FUNCTION "FC_GRP_51" : VOID
TITLE =GROUP =51
{ S7_language := '9(1) Angielski (Stany Zjednoczone)  11.01.2022  09:45:15' }
VERSION : 0.1


VAR_TEMP
  CL : "UDT_CABINET";	//CABINET LOCAL
  CR : "UDT_CABINET";	//CABINET REMOTE
  RelError : BOOL ;	//ERROR RELEASE
  RelErrorCL : BOOL ;	//ERROR RELEASE FROM CABINET LOCAL
  RelErrorCR : BOOL ;	//ERROR RELEASE FROM CABINET REMOTE
  RelControl : BOOL ;	//CONTROL RELEASE
  RelControlCL : BOOL ;	//CONTROL RELEASE FROM CABINET LOCAL
  RelControlCR : BOOL ;	//CONTROL RELEASE FROM CABINET REMOTE
  ErrorConfirm : BOOL ;	//ERROR CONFIRM
  AutoOn : BOOL ;	//AUTOMATIC ON
  AutoOff : BOOL ;	//AUTOMATIC OFF
  RelAuto : BOOL ;	//AUTOMATIC RELEASE
  LAMP_ON : BOOL ;
  TempSetpoint : REAL ;
END_VAR
BEGIN
NETWORK
TITLE =GLOBAL SIGNALS
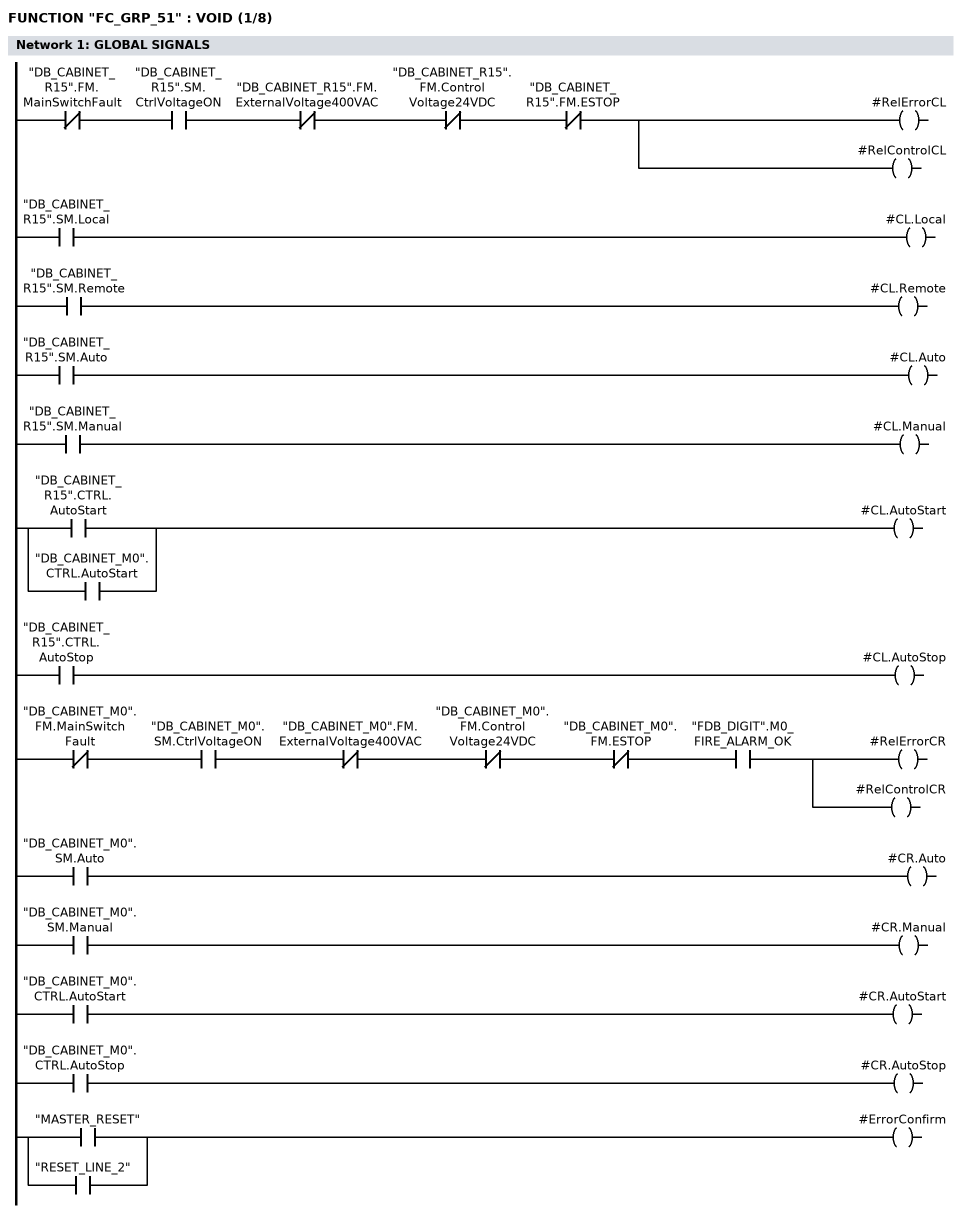
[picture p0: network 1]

//LOCAL
      UN    "DB_CABINET_R15".FM.MainSwitchFault;
      U     "DB_CABINET_R15".SM.CtrlVoltageON;
      UN    "DB_CABINET_R15".FM.ExternalVoltage400VAC;
      UN    "DB_CABINET_R15".FM.ControlVoltage24VDC;
      UN    "DB_CABINET_R15".FM.ESTOP;
      =     #RelErrorCL;
      =     #RelControlCL;

      U     "DB_CABINET_R15".SM.Local;
      =     #CL.Local;
      U     "DB_CABINET_R15".SM.Remote;
      =     #CL.Remote;
      U     "DB_CABINET_R15".SM.Auto;
      =     #CL.Auto;
      U     "DB_CABINET_R15".SM.Manual;
      =     #CL.Manual;
      U     "DB_CABINET_R15".CTRL.AutoStart;
      O     "DB_CABINET_M0".CTRL.AutoStart;
      =     #CL.AutoStart;
      U     "DB_CABINET_R15".CTRL.AutoStop;
      =     #CL.AutoStop;


//REMOTE

      UN    "DB_CABINET_M0".FM.MainSwitchFault;
      U     "DB_CABINET_M0".SM.CtrlVoltageON;
      UN    "DB_CABINET_M0".FM.ExternalVoltage400VAC;
      UN    "DB_CABINET_M0".FM.ControlVoltage24VDC;
//      UN    "DB_CABINET_M0".FM.ControlVoltage230VAC_MS
      UN    "DB_CABINET_M0".FM.ESTOP;
      U     "FDB_DIGIT".M0_FIRE_ALARM_OK;
      =     #RelErrorCR;
      =     #RelControlCR;

      U     "DB_CABINET_M0".SM.Auto;
      =     #CR.Auto;
      U     "DB_CABINET_M0".SM.Manual;
      =     #CR.Manual;
      U     "DB_CABINET_M0".CTRL.AutoStart;
      =     #CR.AutoStart;
      U     "DB_CABINET_M0".CTRL.AutoStop;
      =     #CR.AutoStop;


      U     "MASTER_RESET";
      O     "RESET_LINE_2";
      =     #ErrorConfirm;

NETWORK
TITLE =GLOBAL SIGNALS - GROUP GENERAL ERROR AND WARNING
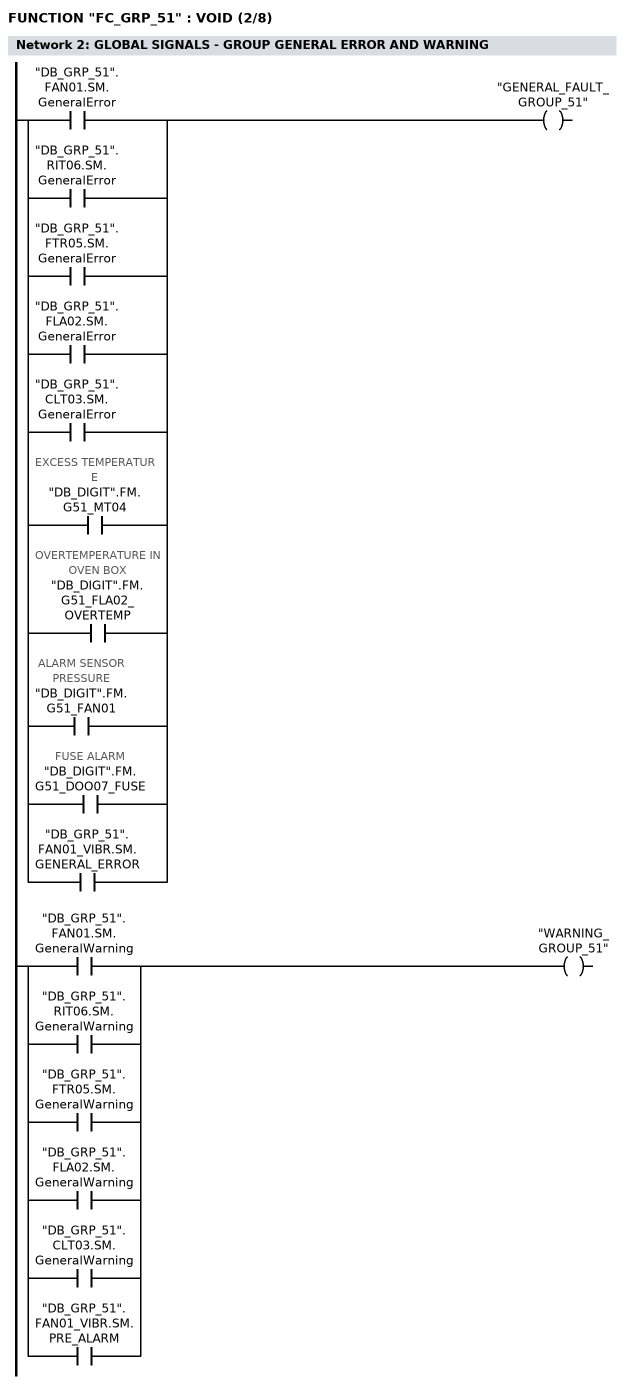
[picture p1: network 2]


      U     "DB_GRP_51".FAN01.SM.GeneralError;
      O     "DB_GRP_51".RIT06.SM.GeneralError;
      O     "DB_GRP_51".FTR05.SM.GeneralError;
      O     "DB_GRP_51".FLA02.SM.GeneralError;
      O     "DB_GRP_51".CLT03.SM.GeneralError;
      O     "DB_DIGIT".FM.G51_MT04; //EXCESS TEMPERATURE
      O     "DB_DIGIT".FM.G51_FLA02_OVERTEMP; //OVERTEMPERATURE IN OVEN BOX
      O     "DB_DIGIT".FM.G51_FAN01; //ALARM SENSOR PRESSURE
      O     "DB_DIGIT".FM.G51_DOO07_FUSE; //FUSE ALARM
      O     "DB_GRP_51".FAN01_VIBR.SM.GENERAL_ERROR;
      =     "GENERAL_FAULT_GROUP_51";

      U     "DB_GRP_51".FAN01.SM.GeneralWarning;
      O     "DB_GRP_51".RIT06.SM.GeneralWarning;
      O     "DB_GRP_51".FTR05.SM.GeneralWarning;
      O     "DB_GRP_51".FLA02.SM.GeneralWarning;
      O     "DB_GRP_51".CLT03.SM.GeneralWarning;
      O     "DB_GRP_51".FAN01_VIBR.SM.PRE_ALARM;
      =     "WARNING_GROUP_51";


NETWORK
TITLE =RELEASE CONTROL
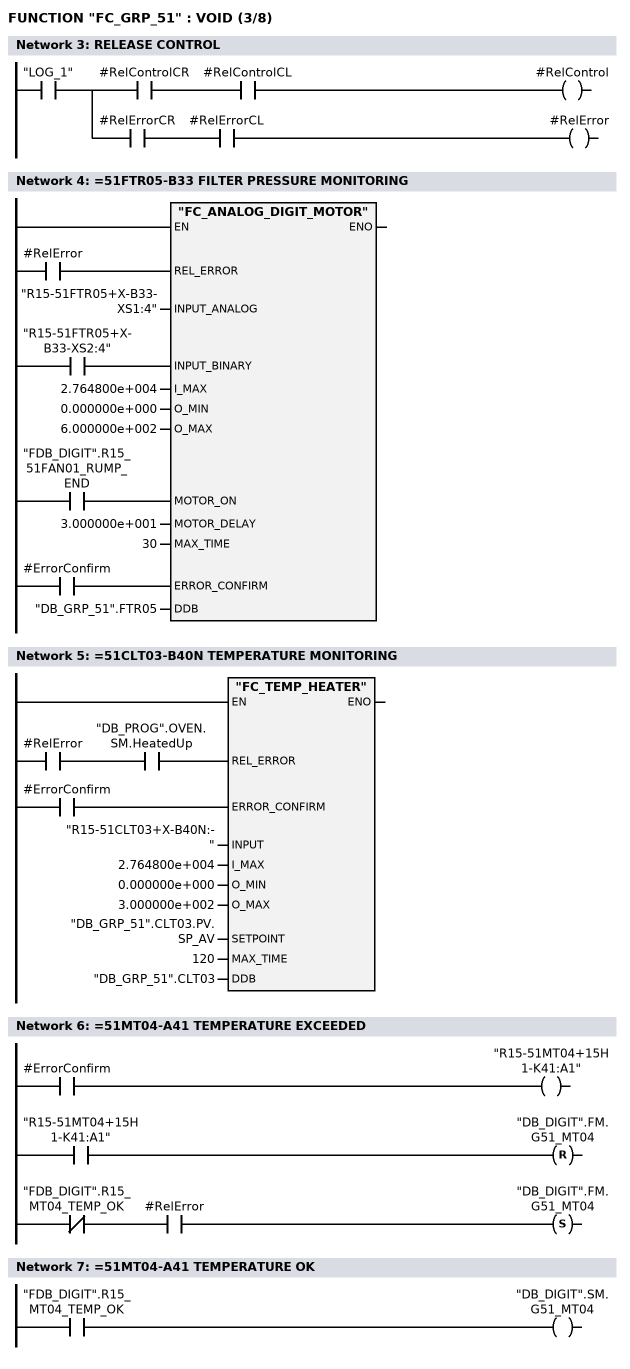
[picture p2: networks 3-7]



      U     "LOG_1";
      =     L     10.0;
      U     L     10.0;
      U     #RelControlCR;
      U     #RelControlCL;
      =     #RelControl;
      U     L     10.0;
      U     #RelErrorCR;
      U     #RelErrorCL;
      =     #RelError;
NETWORK
TITLE ==51FTR05-B33 FILTER PRESSURE MONITORING

      U     #RelError;
      =     L     10.0;
      BLD   103;
      U     "R15-51FTR05+X-B33-XS2:4";
      =     L     10.1;
      BLD   103;
      U     "FDB_DIGIT".R15_51FAN01_RUMP_END;
      =     L     10.2;
      BLD   103;
      U     #ErrorConfirm;
      =     L     10.3;
      BLD   103;
      CALL "FC_ANALOG_DIGIT_MOTOR" (
           REL_ERROR                := L     10.0,
           INPUT_ANALOG             := "R15-51FTR05+X-B33-XS1:4",
           INPUT_BINARY             := L     10.1,
           I_MAX                    := 2.764800e+004,
           O_MIN                    := 0.000000e+000,
           O_MAX                    := 6.000000e+002,
           MOTOR_ON                 := L     10.2,
           MOTOR_DELAY              := 3.000000e+001,
           MAX_TIME                 := 30,
           ERROR_CONFIRM            := L     10.3,
           DDB                      := "DB_GRP_51".FTR05);
      NOP   0;
NETWORK
TITLE ==51CLT03-B40N TEMPERATURE MONITORING

      U     #RelError;
      U     "DB_PROG".OVEN.SM.HeatedUp;
      =     L     10.0;
      BLD   103;
      U     #ErrorConfirm;
      =     L     10.1;
      BLD   103;
      CALL "FC_TEMP_HEATER" (
           REL_ERROR                := L     10.0,
           ERROR_CONFIRM            := L     10.1,
           INPUT                    := "R15-51CLT03+X-B40N:-",
           I_MAX                    := 2.764800e+004,
           O_MIN                    := 0.000000e+000,
           O_MAX                    := 3.000000e+002,
           SETPOINT                 := "DB_GRP_51".CLT03.PV.SP_AV,
           MAX_TIME                 := 120,
           DDB                      := "DB_GRP_51".CLT03);
      NOP   0;
NETWORK
TITLE ==51MT04-A41 TEMPERATURE EXCEEDED

      U     #ErrorConfirm;
      =     "R15-51MT04+15H1-K41:A1";
      U     "R15-51MT04+15H1-K41:A1";
      R     "DB_DIGIT".FM.G51_MT04;
      UN    "FDB_DIGIT".R15_MT04_TEMP_OK;
      U     #RelError;
      S     "DB_DIGIT".FM.G51_MT04;
      NOP   0;
NETWORK
TITLE ==51MT04-A41 TEMPERATURE OK

      U     "FDB_DIGIT".R15_MT04_TEMP_OK;
      =     "DB_DIGIT".SM.G51_MT04;
NETWORK
TITLE ==51DOO07-F1.1 ACCESS DOOR FUSE ERROR
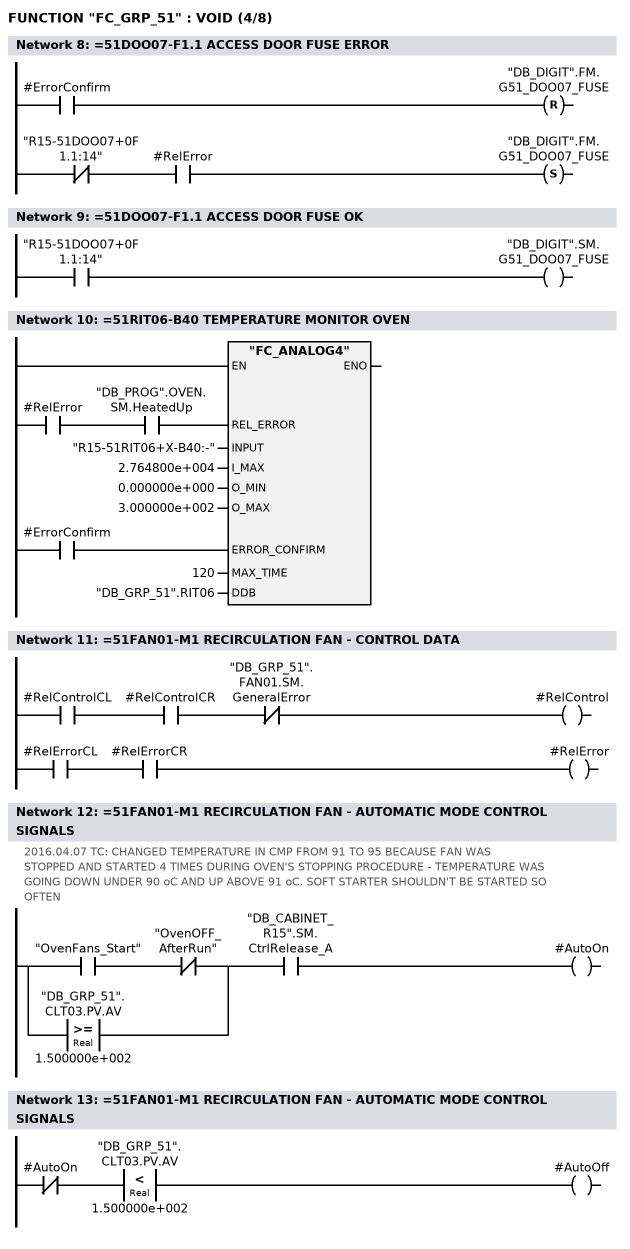
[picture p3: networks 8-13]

      U     #ErrorConfirm;
      R     "DB_DIGIT".FM.G51_DOO07_FUSE;
      UN    "R15-51DOO07+0F1.1:14";
      U     #RelError;
      S     "DB_DIGIT".FM.G51_DOO07_FUSE;
      NOP   0;
NETWORK
TITLE ==51DOO07-F1.1 ACCESS DOOR FUSE OK

      U     "R15-51DOO07+0F1.1:14";
      =     "DB_DIGIT".SM.G51_DOO07_FUSE;
NETWORK
TITLE ==51RIT06-B40 TEMPERATURE MONITOR OVEN

      U     #RelError;
      U     "DB_PROG".OVEN.SM.HeatedUp;
      =     L     10.0;
      BLD   103;
      U     #ErrorConfirm;
      =     L     10.1;
      BLD   103;
      CALL "FC_ANALOG4" (
           REL_ERROR                := L     10.0,
           INPUT                    := "R15-51RIT06+X-B40:-",
           I_MAX                    := 2.764800e+004,
           O_MIN                    := 0.000000e+000,
           O_MAX                    := 3.000000e+002,
           ERROR_CONFIRM            := L     10.1,
           MAX_TIME                 := 120,
           DDB                      := "DB_GRP_51".RIT06);
      NOP   0;
NETWORK
TITLE ==51FAN01-M1 RECIRCULATION FAN - CONTROL DATA

      U     #RelControlCL;
      U     #RelControlCR;
      UN    "DB_GRP_51".FAN01.SM.GeneralError;
      =     #RelControl;


      U     #RelErrorCL;
      U     #RelErrorCR;
      =     #RelError;
NETWORK
TITLE ==51FAN01-M1 RECIRCULATION FAN - AUTOMATIC MODE CONTROL SIGNALS
//2016.04.07 TC: CHANGED TEMPERATURE IN CMP FROM 91 TO 95 BECAUSE FAN WAS
//STOPPED AND STARTED 4 TIMES DURING OVEN'S STOPPING PROCEDURE - TEMPERATURE WAS
//GOING DOWN UNDER 90 oC AND UP ABOVE 91 oC. SOFT STARTER SHOULDN'T BE STARTED SO
//OFTEN
      U(    ;
      U     "OvenFans_Start";
      UN    "OvenOFF_AfterRun";
      O(    ;
      L     "DB_GRP_51".CLT03.PV.AV;
      L     1.500000e+002;
      >=R   ;
      )     ;
      )     ;
      U     "DB_CABINET_R15".SM.CtrlRelease_A;
      =     #AutoOn;
NETWORK
TITLE ==51FAN01-M1 RECIRCULATION FAN - AUTOMATIC MODE CONTROL SIGNALS

      UN    #AutoOn;
      U(    ;
      L     "DB_GRP_51".CLT03.PV.AV;
      L     1.500000e+002;
      <R    ;
      )     ;
      =     #AutoOff;
NETWORK
TITLE ==51FAN01-A1 RECIRCULATION FAN
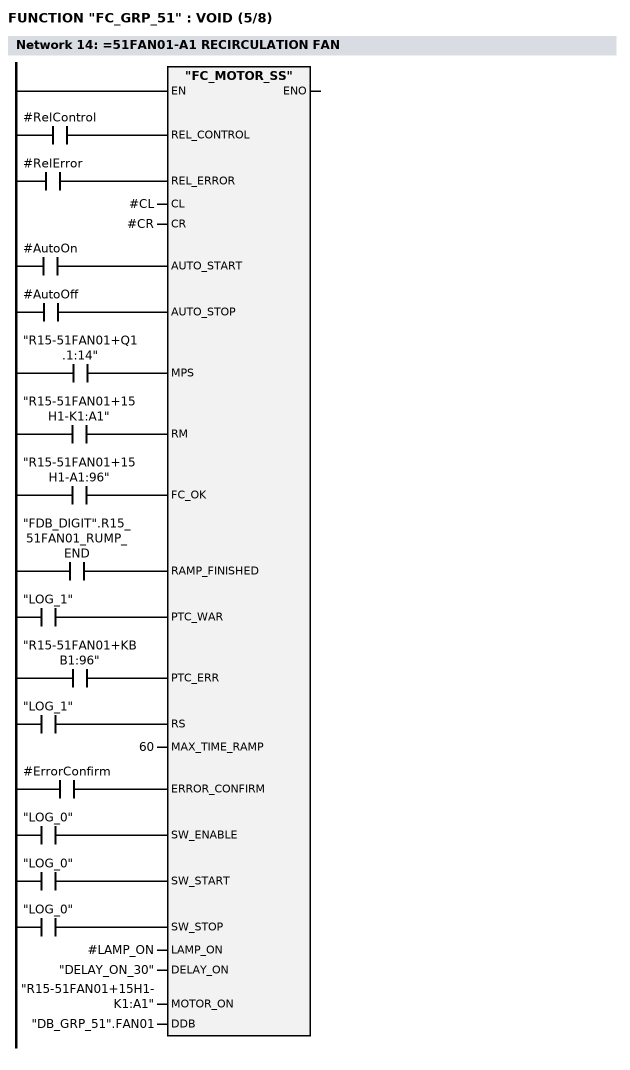
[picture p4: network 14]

      U     #RelControl;
      =     L     10.0;
      BLD   103;
      U     #RelError;
      =     L     10.1;
      BLD   103;
      U     #AutoOn;
      =     L     10.2;
      BLD   103;
      U     #AutoOff;
      =     L     10.3;
      BLD   103;
      U     "R15-51FAN01+Q1.1:14";
      =     L     10.4;
      BLD   103;
      U     "R15-51FAN01+15H1-K1:A1";
      =     L     10.5;
      BLD   103;
      U     "R15-51FAN01+15H1-A1:96";
      =     L     10.6;
      BLD   103;
      U     "FDB_DIGIT".R15_51FAN01_RUMP_END;
      =     L     10.7;
      BLD   103;
      U     "LOG_1";
      =     L     11.0;
      BLD   103;
      U     "R15-51FAN01+KBB1:96";
      =     L     11.1;
      BLD   103;
      U     "LOG_1";
      =     L     11.2;
      BLD   103;
      U     #ErrorConfirm;
      =     L     11.3;
      BLD   103;
      U     "LOG_0";
      =     L     11.4;
      BLD   103;
      U     "LOG_0";
      =     L     11.5;
      BLD   103;
      U     "LOG_0";
      =     L     11.6;
      BLD   103;
      CALL "FC_MOTOR_SS" (
           REL_CONTROL              := L     10.0,
           REL_ERROR                := L     10.1,
           CL                       := #CL,
           CR                       := #CR,
           AUTO_START               := L     10.2,
           AUTO_STOP                := L     10.3,
           MPS                      := L     10.4,
           RM                       := L     10.5,
           FC_OK                    := L     10.6,
           RAMP_FINISHED            := L     10.7,
           PTC_WAR                  := L     11.0,
           PTC_ERR                  := L     11.1,
           RS                       := L     11.2,
           MAX_TIME_RAMP            := 60,
           ERROR_CONFIRM            := L     11.3,
           SW_ENABLE                := L     11.4,
           SW_START                 := L     11.5,
           SW_STOP                  := L     11.6,
           LAMP_ON                  := #LAMP_ON,
           DELAY_ON                 := "DELAY_ON_30",
           MOTOR_ON                 := "R15-51FAN01+15H1-K1:A1",
           DDB                      := "DB_GRP_51".FAN01);
      NOP   0;
NETWORK
TITLE ==51FAN01 - S32F RECIRCULATION FAN PRESSURE OK
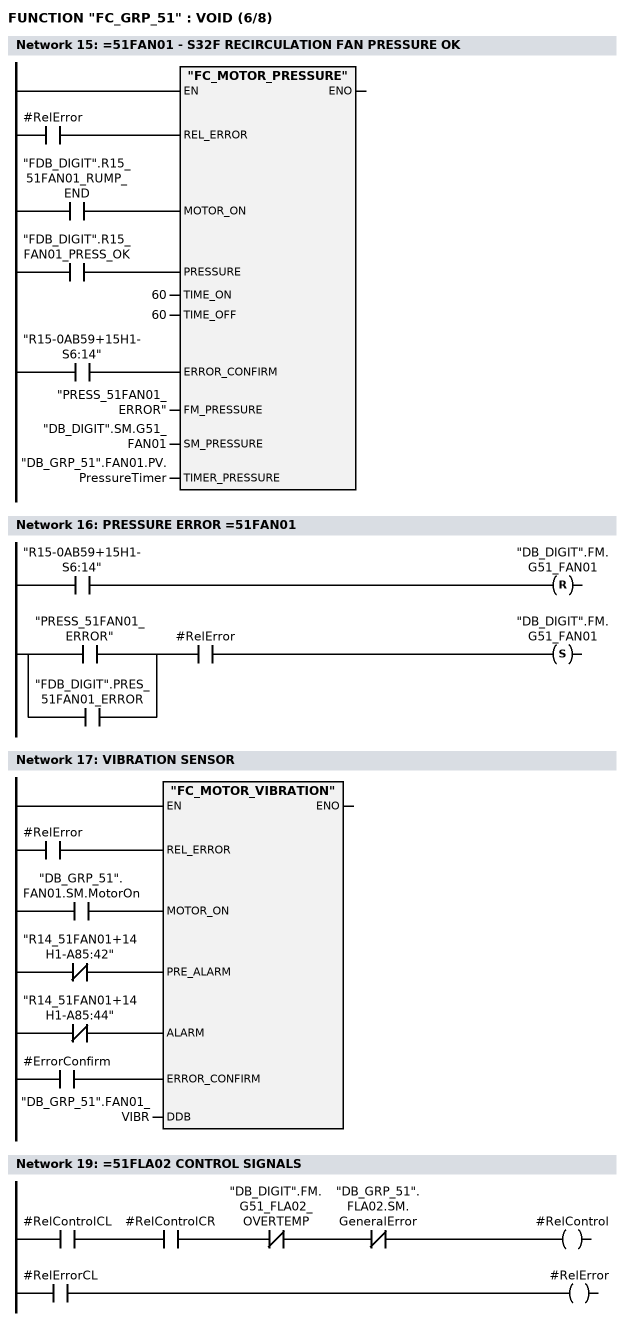
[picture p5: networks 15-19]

      U     #RelError;
      =     L     10.0;
      BLD   103;
      U     "FDB_DIGIT".R15_51FAN01_RUMP_END;
      =     L     10.1;
      BLD   103;
      U     "FDB_DIGIT".R15_FAN01_PRESS_OK;
      =     L     10.2;
      BLD   103;
      U     "R15-0AB59+15H1-S6:14";
      =     L     10.3;
      BLD   103;
      CALL "FC_MOTOR_PRESSURE" (
           REL_ERROR                := L     10.0,
           MOTOR_ON                 := L     10.1,
           PRESSURE                 := L     10.2,
           TIME_ON                  := 60,
           TIME_OFF                 := 60,
           ERROR_CONFIRM            := L     10.3,
           FM_PRESSURE              := "PRESS_51FAN01_ERROR",
           SM_PRESSURE              := "DB_DIGIT".SM.G51_FAN01,
           TIMER_PRESSURE           := "DB_GRP_51".FAN01.PV.PressureTimer);
      NOP   0;
NETWORK
TITLE =PRESSURE ERROR =51FAN01

      U     "R15-0AB59+15H1-S6:14";
      R     "DB_DIGIT".FM.G51_FAN01;
      U(    ;
      O     "PRESS_51FAN01_ERROR";
      O     "FDB_DIGIT".PRES_51FAN01_ERROR;
      )     ;
      U     #RelError;
      S     "DB_DIGIT".FM.G51_FAN01;
      NOP   0;
NETWORK
TITLE =VIBRATION SENSOR

      U     #RelError;
      =     L     10.0;
      BLD   103;
      U     "DB_GRP_51".FAN01.SM.MotorOn;
      =     L     10.1;
      BLD   103;
      UN    "R14_51FAN01+14H1-A85:42";
      =     L     10.2;
      BLD   103;
      UN    "R14_51FAN01+14H1-A85:44";
      =     L     10.3;
      BLD   103;
      U     #ErrorConfirm;
      =     L     10.4;
      BLD   103;
      CALL "FC_MOTOR_VIBRATION" (
           REL_ERROR                := L     10.0,
           MOTOR_ON                 := L     10.1,
           PRE_ALARM                := L     10.2,
           ALARM                    := L     10.3,
           ERROR_CONFIRM            := L     10.4,
           DDB                      := "DB_GRP_51".FAN01_VIBR);
      NOP   0;
NETWORK
TITLE =************ 51FLA02 ****************

NETWORK
TITLE ==51FLA02 CONTROL SIGNALS

      U     #RelControlCL;
      U     #RelControlCR;
      UN    "DB_DIGIT".FM.G51_FLA02_OVERTEMP;
      UN    "DB_GRP_51".FLA02.SM.GeneralError;
      =     #RelControl;


      U     #RelErrorCL;
      =     #RelError;



NETWORK
TITLE ==51FLA02, CONTROL SIGNALS - AUTO_ON
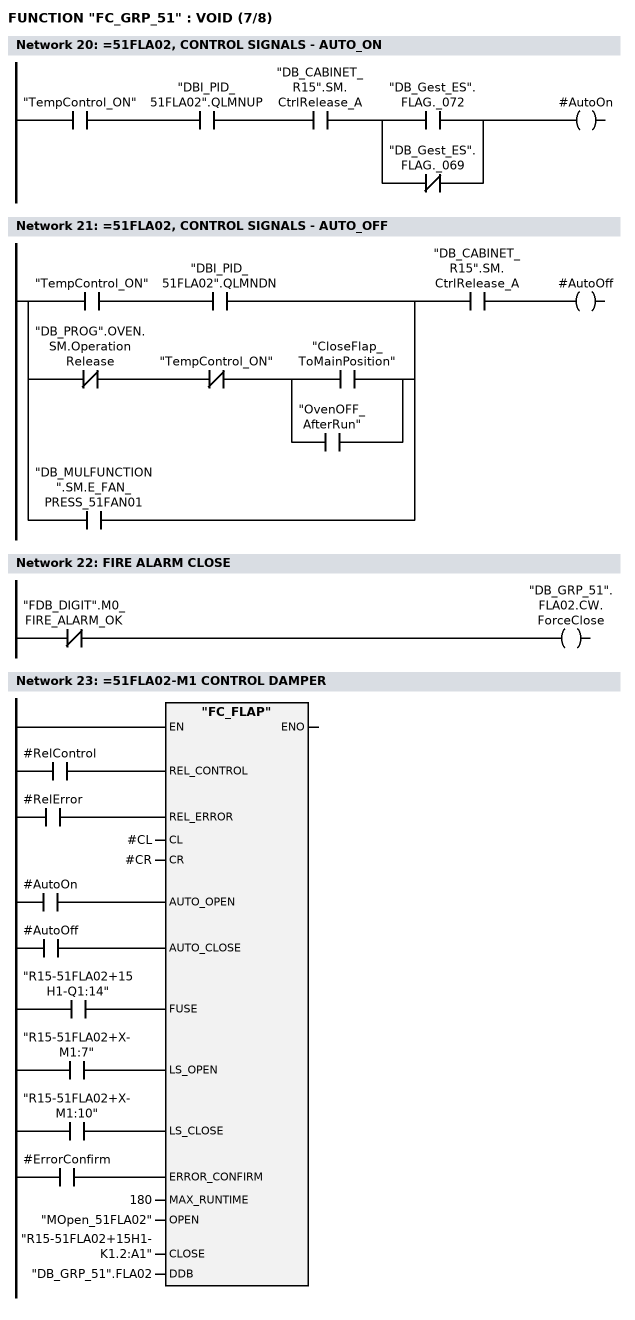
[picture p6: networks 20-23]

      U     "TempControl_ON";
      U     "DBI_PID_51FLA02".QLMNUP;
      U     "DB_CABINET_R15".SM.CtrlRelease_A;
      U(    ;
      O     "DB_Gest_ES".FLAG._072;
      ON    "DB_Gest_ES".FLAG._069;
      )     ;
      =     #AutoOn;
NETWORK
TITLE ==51FLA02, CONTROL SIGNALS - AUTO_OFF

      U(    ;
      U     "TempControl_ON";
      U     "DBI_PID_51FLA02".QLMNDN;
      O     ;
      UN    "DB_PROG".OVEN.SM.OperationRelease;
      UN    "TempControl_ON";
      U(    ;
      O     "CloseFlap_ToMainPosition";
      O     "OvenOFF_AfterRun";
      )     ;
      O     "DB_MULFUNCTION".SM.E_FAN_PRESS_51FAN01;
      )     ;
      U     "DB_CABINET_R15".SM.CtrlRelease_A;
      =     #AutoOff;
NETWORK
TITLE =FIRE ALARM CLOSE

      UN    "FDB_DIGIT".M0_FIRE_ALARM_OK;
      =     "DB_GRP_51".FLA02.CW.ForceClose;
NETWORK
TITLE ==51FLA02-M1 CONTROL DAMPER



      U     #RelControl;
      =     L     10.0;
      BLD   103;
      U     #RelError;
      =     L     10.1;
      BLD   103;
      U     #AutoOn;
      =     L     10.2;
      BLD   103;
      U     #AutoOff;
      =     L     10.3;
      BLD   103;
      U     "R15-51FLA02+15H1-Q1:14";
      =     L     10.4;
      BLD   103;
      U     "R15-51FLA02+X-M1:7";
      =     L     10.5;
      BLD   103;
      U     "R15-51FLA02+X-M1:10";
      =     L     10.6;
      BLD   103;
      U     #ErrorConfirm;
      =     L     10.7;
      BLD   103;
      CALL "FC_FLAP" (
           REL_CONTROL              := L     10.0,
           REL_ERROR                := L     10.1,
           CL                       := #CL,
           CR                       := #CR,
           AUTO_OPEN                := L     10.2,
           AUTO_CLOSE               := L     10.3,
           FUSE                     := L     10.4,
           LS_OPEN                  := L     10.5,
           LS_CLOSE                 := L     10.6,
           ERROR_CONFIRM            := L     10.7,
           MAX_RUNTIME              := 180,
           OPEN                     := "MOpen_51FLA02",
           CLOSE                    := "R15-51FLA02+15H1-K1.2:A1",
           DDB                      := "DB_GRP_51".FLA02);
      NOP   0;
NETWORK
TITLE =MANUAL INTERLOCKS - OPEN 43FLA02
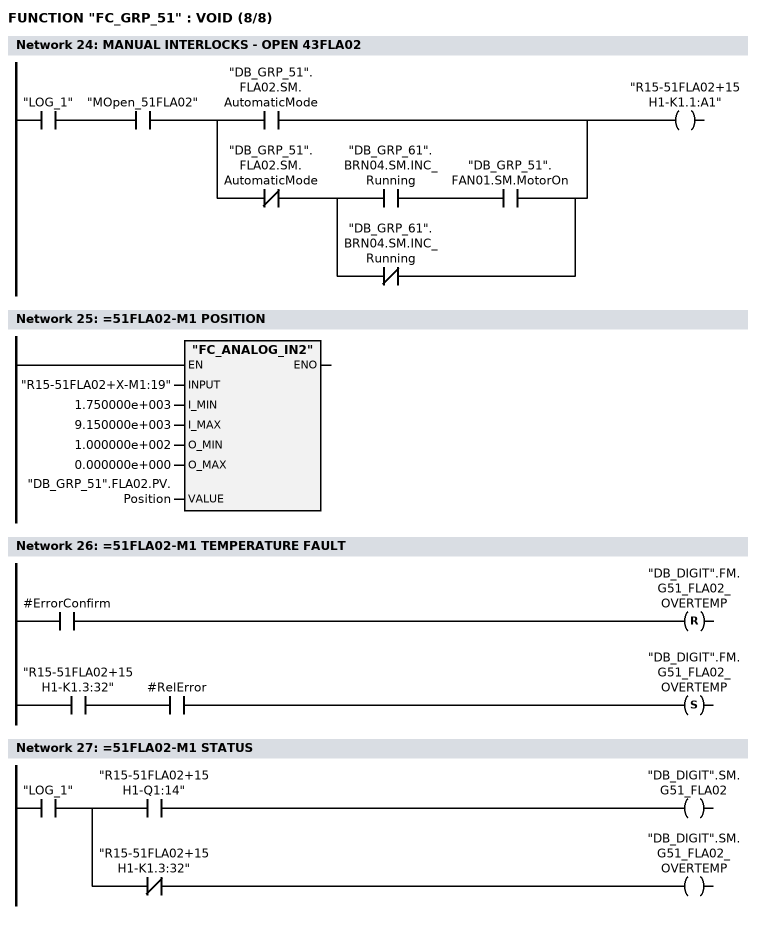
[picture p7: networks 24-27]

      U     "LOG_1";
      U     "MOpen_51FLA02";
      U(    ;
      O     "DB_GRP_51".FLA02.SM.AutomaticMode;
      O     ;
      UN    "DB_GRP_51".FLA02.SM.AutomaticMode;
      U(    ;
      U     "DB_GRP_61".BRN04.SM.INC_Running;
      U     "DB_GRP_51".FAN01.SM.MotorOn;
      ON    "DB_GRP_61".BRN04.SM.INC_Running;
      )     ;
      )     ;
      =     "R15-51FLA02+15H1-K1.1:A1";
NETWORK
TITLE ==51FLA02-M1 POSITION

      CALL "FC_ANALOG_IN2" (
           INPUT                    := "R15-51FLA02+X-M1:19",
           I_MIN                    := 1.750000e+003,
           I_MAX                    := 9.150000e+003,
           O_MIN                    := 1.000000e+002,
           O_MAX                    := 0.000000e+000,
           VALUE                    := "DB_GRP_51".FLA02.PV.Position);
      NOP   0;
NETWORK
TITLE ==51FLA02-M1 TEMPERATURE FAULT

      U     #ErrorConfirm;
      R     "DB_DIGIT".FM.G51_FLA02_OVERTEMP;
      U     "R15-51FLA02+15H1-K1.3:32";
      U     #RelError;
      S     "DB_DIGIT".FM.G51_FLA02_OVERTEMP;
      NOP   0;
NETWORK
TITLE ==51FLA02-M1 STATUS

      U     "LOG_1";
      =     L     10.0;
      U     L     10.0;
      U     "R15-51FLA02+15H1-Q1:14";
      =     "DB_DIGIT".SM.G51_FLA02;
      U     L     10.0;
      UN    "R15-51FLA02+15H1-K1.3:32";
      =     "DB_DIGIT".SM.G51_FLA02_OVERTEMP;
NETWORK
TITLE =END

END_FUNCTION

